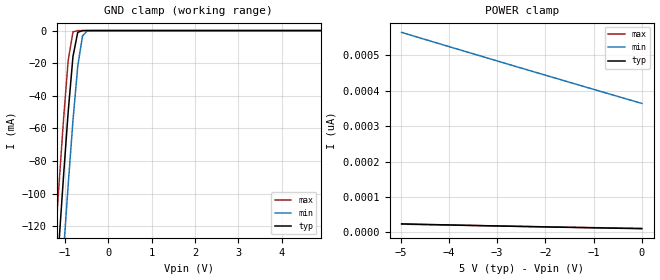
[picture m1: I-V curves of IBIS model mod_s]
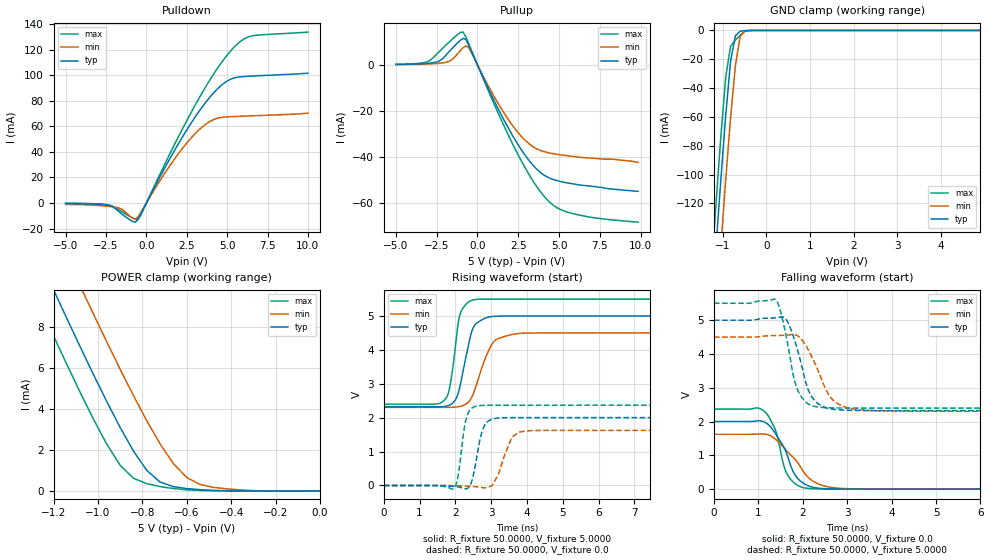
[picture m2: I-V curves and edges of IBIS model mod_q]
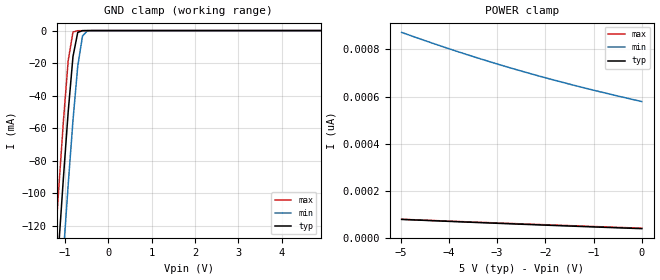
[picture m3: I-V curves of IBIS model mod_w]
| IBIS (I/O, Buffer, Information, Specification) Model, officially
| electronic behavioral standard for Buffer structures of digital pins.
[IBIS ver]  4.0
[File name] model_g9_tssop8.ibs
[File Rev]  1.0
[Date]   17 Sep 2015
[Source]   CAD & Design Services (Catania) - STMicroelectronics
[Notes]
  (Note1)  This IBIS model includes the TSSOP8 ceramic package parasitic data
  (Note2)  This IBIS model considers: VCC= 5.0(TYP), 4.50(MIN), 5.50(MAX)
  (Note3)  This IBIS model has some Notes about the non-monotonicity
   of the I-V curves, but they are not indicative of problems
   inside the model;
[Copyright] (c) 2015 STMicroelectronics
|   Component M95XXX
[Component] M95XXX
[Manufacturer] STMicroelectronics
[Package]
| variable   typ   min   max
R_pkg   0.0   0.0   0.0
L_pkg   0.0H   0.0H   0.0H
C_pkg   0.0F   0.0F   0.0F
[Pin]   signal_name   model_name   R_pin   L_pin   C_pin
1   SN   mod_s   NA   NA   NA
2   Q   mod_q   NA   NA   NA
3   WN   mod_w   NA   NA   NA
4   GND   GND   NA   NA   NA
5   D   mod_s   NA   NA   NA
6   C   mod_s   NA   NA   NA
7   HOLDN   mod_h   NA   NA   NA
8   VCC   POWER   NA   NA   NA
[Package Model]  182696_TSSOP8
[Define Package Model]  182696_TSSOP8
[Manufacturer]  STMicroelectronics
[OEM]  STMicroelectronics
[Description]  8 pin TSSOP package
[Number Of Pins]  8
[Pin Numbers]
|Pin Num   Terminal Name
1   | net1
2   | net2
3   | net3
4   | net4_GND
5   | net5
6   | net6
7   | net7
8   | net8_VDD
[Model Data]
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[End Model Data]
[End Package Model]
| Models and submodels in the file (4): mod_s (Input), mod_q (I/O), mod_w (Input), mod_h (Input)
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|   Model mod_s
[Model]   mod_s
Model_type Input
Vinl   =   1.500V
Vinh   =   3.500V
C_comp   2.120pF   2.024pF   2.323pF
[Temperature Range]   25.0000   0.1050k   -40.0000
[Voltage Range]   5.0000V   4.5000V   5.5000V
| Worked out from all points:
|   GND clamp passes 1 mA (typ) near -0.70 V on its own axis
[GND_clamp]
|Voltage   I(typ)   I(min)   I(max)
-5V       -1.764A    -1.807A    -1.733A
-1.26V    -176.7mA   -223.6mA   -141.2mA
-1.15V    -132.7mA   -179.4mA   -97.27mA
-1.04V    -89.88mA   -136.2mA   -55.14mA
-930mV    -49.58mA   -94.31mA   -18.16mA
-820mV    -15.87mA   -55.06mA   -757uA
-710mV    -1.068mA   -21.8mA    -5.45uA
-600mV    -23.1uA    -3.301mA   -36.27nA
-490mV    -459.2nA   -183.8uA   -242.2pA
4.9V      10.56pA    379.5pA    10.13pA
[POWER_clamp]
|Voltage   I(typ)   I(min)   I(max)
-4.98V    24.27pA    563.8pA    23.46pA
-3.96V    21.17pA    522.2pA    20.77pA
-2.64V    17.45pA    468.9pA    17.5pA
0V        10.79pA    363.7pA    11.44pA
|   Model mod_q
[Model]   mod_q
Model_type I/O
Polarity   Non-Inverting
Enable   Active-Low
Vinl   =   1.500V
Vinh   =   3.500V
Vmeas  =   2.500V
Cref   =   30pF
C_comp   2.793pF   2.547pF   3.063pF
[Temperature Range]   25.0000   0.1050k   -40.0000
[Voltage Range]   5.0000V   4.5000V   5.5000V
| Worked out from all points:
|   slope of the pulldown table from 0 to 0.75 V, typ, clamps not added: 41 ohm
|   slope of the pullup table from 0 to 0.75 V, typ, clamps not added: 64.9 ohm
|   GND clamp passes 1 mA (typ) near -0.62 V on its own axis
|   POWER clamp passes 1 mA (typ) near -0.78 V on its own axis
|   rising waveform, R_fixture 50.0000, V_fixture 5.0000: 20-80 % time 323ps typ, 451ps min, 232ps max; typ from 2.32 V to 5 V
|   rising waveform, R_fixture 50.0000, V_fixture 0.0: 20-80 % time 227ps typ, 334ps min, 180ps max; typ from 0 V to 2 V
|   falling waveform, R_fixture 50.0000, V_fixture 0.0: 20-80 % time 432ps typ, 619ps min, 304ps max; typ from 2 V to 0 V
|   falling waveform, R_fixture 50.0000, V_fixture 5.0000: 20-80 % time 348ps typ, 462ps min, 290ps max; typ from 5 V to 2.32 V
[Pulldown]
|Voltage   I(typ)   I(min)   I(max)
-5V       -504uA     -1.11mA    -42.1uA
-2.28V    -2mA       -2.8mA     -1.8mA
-1.48V    -9mA       -5.2mA     -7.1mA
-840mV    -14.57mA   -11.91mA   -11.84mA
-520mV    -12.8mA    -10.9mA    -12.96mA
1.4V      33.44mA    28.24mA    37.15mA
2.84V     63.92mA    51.88mA    72.48mA
4.12V     85.6mA     65.04mA    100.1mA
5.24V     97.05mA    67.58mA    119.4mA
5.88V     98.83mA    67.92mA    127mA
6.52V     99.34mA    68.23mA    130.8mA
10V       101.6mA    70.3mA     133.8mA
[Pullup]
|Voltage   I(typ)   I(min)   I(max)
-5V       220uA      160uA      270uA
-3.12V    642uA      389uA      1.259mA
-2.48V    1.34mA     622uA      4.783mA
-1.68V    6.188mA    1.768mA    10.3mA
-880mV    11.53mA    7.454mA    14.28mA
-560mV    8.919mA    7.757mA    9.648mA
1.04V     -15.82mA   -13.96mA   -17.33mA
2.32V     -32.77mA   -27.98mA   -36.74mA
3.28V     -42.61mA   -34.96mA   -49.1mA
4.24V     -48.6mA    -38.01mA   -58.41mA
5.84V     -51.71mA   -39.8mA    -64.67mA
9.84V     -55mA      -42.4mA    -68.4mA
[GND_clamp]
|Voltage   I(typ)   I(min)   I(max)
-5V       -1.918A    -1.959A    -1.89A
-1.26V    -196.9mA   -243.3mA   -166.6mA
-1.15V    -149.1mA   -195.5mA   -118.8mA
-1.04V    -102.6mA   -148.7mA   -72.9mA
-930mV    -58.74mA   -103.3mA   -32.17mA
-820mV    -21.58mA   -60.77mA   -11.08mA
-710mV    -3.653mA   -24.61mA   -6.723mA
-600mV    -555.3uA   -4.188mA   -3.311mA
-490mV    -79.08uA   -422uA     -612.8uA
-380mV    -6.392uA   -66.67uA   -6.411uA
4.9V      216.5pA    85.29uA    174.3pA
[POWER_clamp]
|Voltage   I(typ)   I(min)   I(max)
-4.98V    102.8mA    105.6mA    100.8mA
-1.32V    12.64mA    15.62mA    10.38mA
-1.26V    11.22mA    14.2mA     8.958mA
-1.2V     9.805mA    12.79mA    7.55mA
-1.08V    7.024mA    9.991mA    4.803mA
-1.02V    5.669mA    8.614mA    3.493mA
-960mV    4.351mA    7.259mA    2.274mA
-840mV    1.942mA    4.644mA    616.9uA
-720mV    429.6uA    2.288mA    210.9uA
-600mV    115.4uA    653.4uA    55.12uA
-420mV    9.884uA    103.2uA    932.9nA
0V        230.6pA    2.069nA    241.5pA
[Ramp]
| variable   typ   min   max
dV/dt_r  1.2015/0.2702n   0.9748/0.3575n   1.4213/0.2190n
dV/dt_f  1.6073/0.3921n   1.3163/0.5122n   1.8614/0.3216n
R_load = 50.0000
[Rising Waveform]
R_fixture= 50.0000
V_fixture= 5.0000
V_fixture_min= 4.5000
V_fixture_max= 5.5000
|time   V(typ)   V(min)   V(max)
0s        2.323V     2.304V     2.398V
1.485ns   2.322V     2.304V     2.405V
1.725ns   2.336V     2.304V     2.556V
1.875ns   2.393V     2.305V     3.095V
2.115ns   2.868V     2.329V     4.988V
2.265ns   3.637V     2.384V     5.309V
2.505ns   4.671V     2.717V     5.477V
3.045ns   4.987V     4.204V     5.5V
3.675ns   5V         4.473V     5.5V
15ns      5V         4.5V       5.5V
[Rising Waveform]
R_fixture= 50.0000
V_fixture= 0.0
V_fixture_min= 0.0
V_fixture_max= 0.0
|time   V(typ)   V(min)   V(max)
0s        7.837nV    247.1nV    7.911nV
1.95ns    -26.74mV   -5.065mV   -97.76mV
2.07ns    -42.23mV   -7.666mV   243.6mV
2.295ns   -101.5mV   -18.87mV   1.941V
2.46ns    137.3mV    -28.3mV    2.281V
2.64ns    1.096V     -45.47mV   2.351V
2.94ns    1.915V     -36.83mV   2.367V
3.57ns    2.002V     1.403V     2.368V
3.99ns    2.002V     1.611V     2.368V
15ns      2.002V     1.625V     2.368V
[Falling Waveform]
R_fixture= 50.0000
V_fixture= 0.0
V_fixture_min= 0.0
V_fixture_max= 0.0
|time   V(typ)   V(min)   V(max)
0s        2.002V     1.624V     2.368V
1.14ns    1.983V     1.631V     2.296V
1.38ns    1.653V     1.484V     1.765V
1.56ns    1.279V     1.246V     755.4mV
1.65ns    1.009V     1.117V     442.2mV
1.83ns    413mV      876.4mV    159.7mV
2.1ns     113.9mV    378.9mV    25.53mV
2.49ns    16.17mV    93.26mV    3.664mV
3.15ns    1.482mV    9.06mV     174.9uV
15ns      -21.19nV   212.7nV    11.89nV
[Falling Waveform]
R_fixture= 50.0000
V_fixture= 5.0000
V_fixture_min= 4.5000
V_fixture_max= 5.5000
|time   V(typ)   V(min)   V(max)
0s        5V         4.5V       5.5V
1.41ns    5.072V     4.545V     5.577V
1.62ns    5.028V     4.556V     4.562V
1.86ns    4.215V     4.553V     3.016V
2.1ns     3.02V      4.178V     2.543V
2.31ns    2.567V     3.614V     2.436V
2.55ns    2.398V     2.869V     2.41V
2.7ns     2.362V     2.615V     2.405V
3.42ns    2.326V     2.333V     2.399V
15ns      2.323V     2.304V     2.398V
|   Model mod_w
[Model]   mod_w
Model_type Input
Vinl   =   1.500V
Vinh   =   3.500V
C_comp   2.120pF   2.024pF   2.323pF
[Temperature Range]   25.0000   0.1050k   -40.0000
[Voltage Range]   5.0000V   4.5000V   5.5000V
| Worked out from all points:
|   GND clamp passes 1 mA (typ) near -0.70 V on its own axis
[GND_clamp]
|Voltage   I(typ)   I(min)   I(max)
-5V       -1.766A    -1.808A    -1.734A
-1.26V    -176.9mA   -223.8mA   -141.5mA
-1.15V    -132.9mA   -179.6mA   -97.5mA
-1.04V    -90.04mA   -136.3mA   -55.33mA
-930mV    -49.7mA    -94.42mA   -18.31mA
-820mV    -15.96mA   -55.14mA   -879.8uA
-710mV    -1.123mA   -21.85mA   -94.22uA
-600mV    -50.36uA   -3.331mA   -55.9uA
-490mV    -8.761uA   -198.4uA   -25.47uA
4.9V      37.72pA    597.7pA    35.95pA
[POWER_clamp]
|Voltage   I(typ)   I(min)   I(max)
-4.98V    77.79pA    872.7pA    78.35pA
-4.26V    71.63pA    821.2pA    72.58pA
-3.66V    66.63pA    780.6pA    67.85pA
-3.12V    62.23pA    746pA      63.65pA
-2.58V    57.92pA    713.2pA    59.5pA
-1.98V    53.24pA    678.8pA    54.95pA
-1.44V    49.11pA    649.7pA    50.9pA
-840mV    44.61pA    619.1pA    46.46pA
0V        38.45pA    578.7pA    40.3pA
